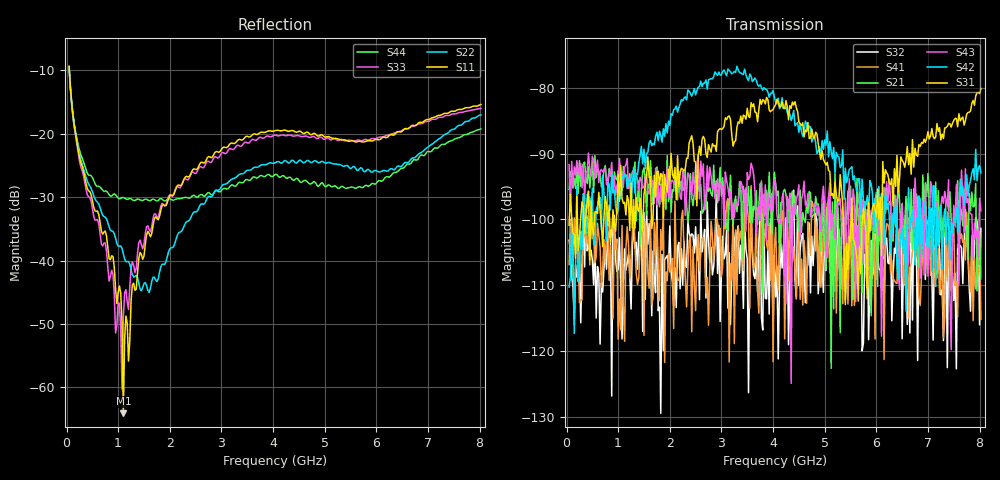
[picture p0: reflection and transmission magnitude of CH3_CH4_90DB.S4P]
!Agilent Technologies,E5071C,MY46316741,A.11.02
!Date: Thu May 28 14:59:53 2026
!Data & Calibration Information:
!1:CH3 INPUT 2:CH3 OUTPUT 3:CH4 INPUT 4:CH4 OUTPUT
!Freq	S11:SOLT4(ON)	S12:SOLT4(ON)	S13:SOLT4(ON)	S14:SOLT4(ON)
!	S21:SOLT4(ON)	S22:SOLT4(ON)	S23:SOLT4(ON)	S24:SOLT4(ON)
!	S31:SOLT4(ON)	S32:SOLT4(ON)	S33:SOLT4(ON)	S34:SOLT4(ON)
!	S41:SOLT4(ON)	S42:SOLT4(ON)	S43:SOLT4(ON)	S44:SOLT4(ON)
!PortZ  Port1:50+j0  Port2:50+j0  Port3:50+j0  Port4:50+j0
!Above PortZ is port z conversion or system Z0 setting when saving the data.
!When reading, reference impedance value at option line is always used.
# Hz S dB R 50
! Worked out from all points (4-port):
!   320 points, 50 MHz to 8.025 GHz, reference 50 ohm
!   strongest paths, dB at 50 MHz, 2.05 GHz, 4.05 GHz, 6.05 GHz, 8.025 GHz:
!     S31: -100.9, -93.1, -82.6, -100.1, -80.1
!     S42: -110.3, -84.2, -82.2, -95.0, -92.9
!     S43: -91.7, -94.0, -94.6, -102.4, -98.7
!     S21: -95.5, -95.5, -94.7, -96.2, -109.0
!     S41: -106.9, -105.9, -101.2, -102.1, -115.2
!     S32: -103.2, -109.5, -111.8, -107.5, -101.4
!   lowest |S11| = -64.1 dB at 1.1 GHz (marker M1), VSWR 1.00, Z = 50 + j0.062 ohm
!   |S11| at or under -10 dB: 55.06 MHz to end of sweep
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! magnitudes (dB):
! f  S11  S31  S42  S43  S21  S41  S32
! 50 MHz  -9.3  -100.9  -110.3  -91.7  -95.5  -106.9  -103.2
! 1.05 GHz  -45.2  -91.8  -96.9  -93.0  -92.5  -116.8  -110.0
! 1.1 GHz  -64.1  -97.6  -93.8  -95.1  -92.0  -113.0  -110.7
! 1.15 GHz  -48.8  -99.3  -93.4  -91.7  -93.5  -104.4  -107.7
! 1.425 GHz  -38.7  -96.8  -90.3  -93.6  -104.0  -104.3  -101.7
! 2.6 GHz  -24.5  -90.3  -79.0  -91.1  -94.7  -105.4  -98.8
! 8.025 GHz  -15.4  -80.1  -92.9  -98.7  -109.0  -115.2  -101.4
